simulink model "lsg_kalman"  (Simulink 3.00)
settings: Solver=ode45  StartTime=0.0  StopTime=Tstop  MaxStep=max_step  RelTol=1e-3
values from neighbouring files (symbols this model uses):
  den = [0.02 1]    [lsg_regelung_ini.m]    (also in lsg_system_ini.m; lsg_sys_kalman_ini.m; system_ini.m; sys_kalman_ini.m)
  g = 2    [lsg_regelung_ini.m]    (also in lsg_system_ini.m; lsg_sys_kalman_ini.m; system_ini.m; sys_kalman_ini.m)
  num = 2    [lsg_regelung_ini.m]    (also in lsg_system_ini.m; lsg_sys_kalman_ini.m; system_ini.m; sys_kalman_ini.m)
  p = [-2 -3+10*i -3-10*i]    [lsg_regelung_ini.m]    (also in lsg_system_ini.m; lsg_sys_kalman_ini.m; system_ini.m; sys_kalman_ini.m)
  Q = 1e-3    (= 0.001)    [lsg_regelung_ini.m]    (also in lsg_sys_kalman_ini.m; sys_kalman_ini.m = 1e-06)
  R = 1e-3    (= 0.001)    [lsg_regelung_ini.m]    (also in lsg_sys_kalman_ini.m; sys_kalman_ini.m = 1e-06)
  verst = 100    [lsg_regelung_ini.m]    (also in lsg_system_ini.m; lsg_sys_kalman_ini.m; system_ini.m; sys_kalman_ini.m)
  z = [1 1]    [lsg_regelung_ini.m]    (also in lsg_system_ini.m; lsg_sys_kalman_ini.m; system_ini.m; sys_kalman_ini.m)
undefined symbols (not defined in the file or in its folder): kest

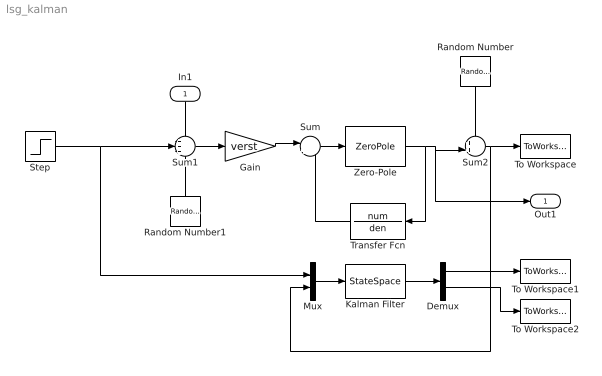
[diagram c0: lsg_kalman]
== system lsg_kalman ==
  In1 : Inport  Orientation=down  Port=1  PortWidth=-1  SampleTime=-1  DataType=auto
  Demux : Demux  Outputs=[1 4]
  Gain : Gain  Gain=verst  SaturateOnIntegerOverflow=on
  Kalman Filter : StateSpace  A=kest.a  B=kest.b  C=kest.c  D=kest.d  X0=0
  Mux : Mux  Inputs=2
  Random Number : RandomNumber  Orientation=down  Mean=0  Variance=R  Seed=0  SampleTime=0
  Random Number1 : RandomNumber  Orientation=up  Mean=0  Variance=Q  Seed=0  SampleTime=0
  Step : Step  Time=1  Before=0  After=1  SampleTime=0
  Sum : Sum  Inputs=|++  SaturateOnIntegerOverflow=on
  Sum1 : Sum  Inputs=+++  SaturateOnIntegerOverflow=on
  Sum2 : Sum  Inputs=++|  SaturateOnIntegerOverflow=on
  To Workspace : ToWorkspace  VariableName=y  SampleTime=-1  SaveFormat=Matrix
  To Workspace1 : ToWorkspace  VariableName=ye  SampleTime=-1  SaveFormat=Matrix
  To Workspace2 : ToWorkspace  VariableName=xe  SampleTime=-1  SaveFormat=Matrix
  Transfer Fcn : TransferFcn  Orientation=left  Numerator=num  Denominator=den
  Zero-Pole : ZeroPole  Zeros=z  Poles=p  Gain=g
  Out1 : Outport  Port=1
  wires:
  Transfer Fcn/1 -> Sum/2
  Sum/1 -> Zero-Pole/1
  Gain/1 -> Sum/1
  Zero-Pole/1 -> Transfer Fcn/1, Sum2/2, Out1/1
  Random Number/1 -> Sum2/1
  Sum2/1 -> To Workspace/1, Mux/2
  In1/1 -> Sum1/1
  Random Number1/1 -> Sum1/3
  Sum1/1 -> Gain/1
  Mux/1 -> Kalman Filter/1
  Step/1 -> Sum1/2, Mux/1
  Kalman Filter/1 -> Demux/1
  Demux/1 -> To Workspace1/1
  Demux/2 -> To Workspace2/1
